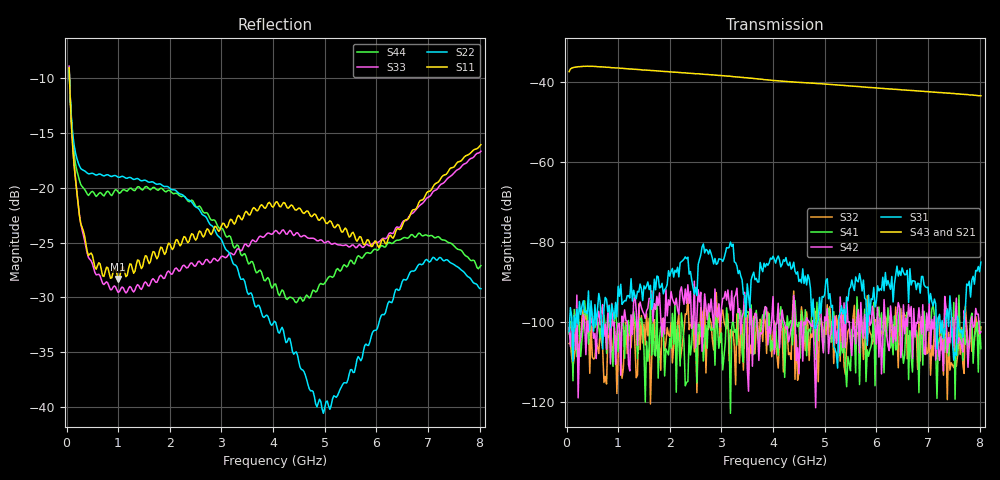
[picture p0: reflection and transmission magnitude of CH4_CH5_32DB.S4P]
!Agilent Technologies,E5071C,MY46316741,A.11.02
!Date: Mon Jun 01 11:46:56 2026
!Data & Calibration Information:
!1:CH4 INPUT 2:CH4 OUTPUT 3:CH5 INPUT 4:CH5 OUTPUT
!Freq	S11:SOLT4(ON)	S12:SOLT4(ON)	S13:SOLT4(ON)	S14:SOLT4(ON)
!	S21:SOLT4(ON)	S22:SOLT4(ON)	S23:SOLT4(ON)	S24:SOLT4(ON)
!	S31:SOLT4(ON)	S32:SOLT4(ON)	S33:SOLT4(ON)	S34:SOLT4(ON)
!	S41:SOLT4(ON)	S42:SOLT4(ON)	S43:SOLT4(ON)	S44:SOLT4(ON)
!PortZ  Port1:50+j0  Port2:50+j0  Port3:50+j0  Port4:50+j0
!Above PortZ is port z conversion or system Z0 setting when saving the data.
!When reading, reference impedance value at option line is always used.
# Hz S dB R 50
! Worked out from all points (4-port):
!   320 points, 50 MHz to 8.025 GHz, reference 50 ohm
!   strongest paths, dB at 50 MHz, 2.05 GHz, 4.05 GHz, 6.05 GHz, 8.025 GHz:
!     S43: -37.4, -37.5, -39.7, -41.6, -43.4
!     S21: -37.5, -37.6, -39.8, -41.7, -43.7
!     S31: -102.3, -86.6, -85.2, -92.2, -85.0
!     S42: -101.4, -94.2, -100.7, -108.7, -102.4
!     S41: -102.9, -97.8, -100.4, -96.2, -106.6
!     S32: -105.3, -110.2, -105.9, -102.7, -101.2
!   lowest |S11| = -28.3 dB at 1 GHz (marker M1), VSWR 1.08, Z = 47.7 - j2.99 ohm
!   |S11| at or under -10 dB: 57.17 MHz to end of sweep
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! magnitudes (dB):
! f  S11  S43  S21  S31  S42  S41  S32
! 50 MHz  -9.1  -37.4  -37.5  -102.3  -101.4  -102.9  -105.3
! 275 MHz  -23.3  -36.2  -36.2  -98.1  -104.0  -108.6  -104.0
! 1 GHz  -28.3  -36.5  -36.6  -91.0  -100.4  -107.4  -108.4
! 2.7 GHz  -24.0  -38.1  -38.2  -81.8  -96.0  -100.8  -112.7
! 4.975 GHz  -22.8  -40.5  -40.7  -93.8  -107.6  -107.3  -104.5
! 6.825 GHz  -21.4  -42.3  -42.5  -90.3  -96.4  -117.6  -99.8
! 8.025 GHz  -16.1  -43.4  -43.7  -85.0  -102.4  -106.6  -101.2
